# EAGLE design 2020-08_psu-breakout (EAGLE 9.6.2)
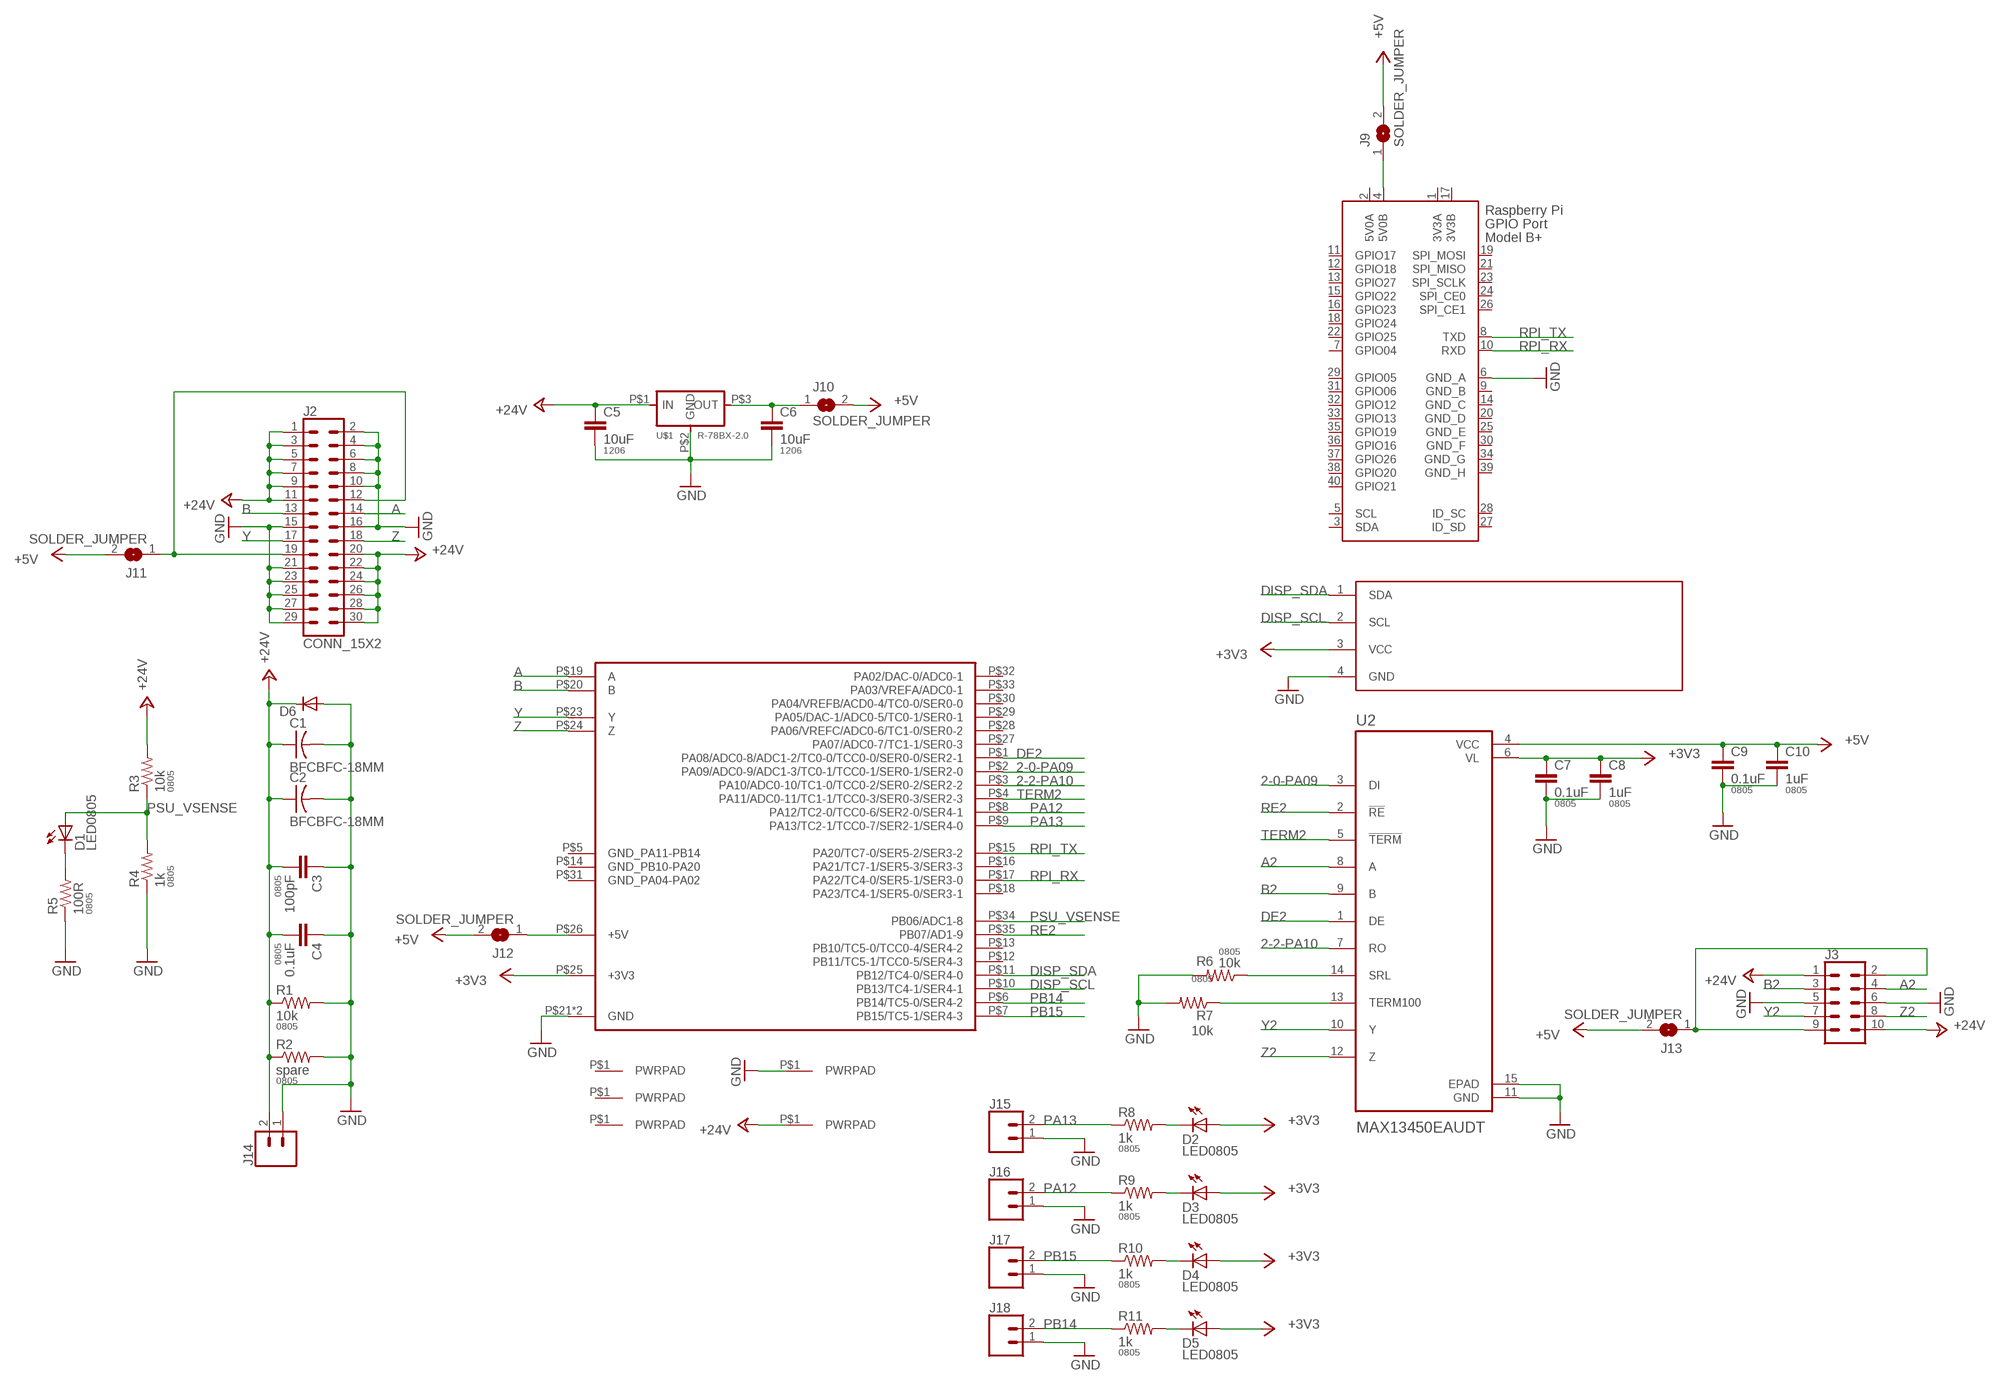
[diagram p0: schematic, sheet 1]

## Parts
C1  BFCBFC-18MM  [BFC-18MM-7-5MM]
C2  BFCBFC-18MM  [BFC-18MM-7-5MM]
C3  100pF  CAP0805  [0805]
C4  0.1uF  CAP0805  [0805]
C5  10uF  CAP1206  [1206]
C6  10uF  CAP1206  [1206]
C7  0.1uF  CAP0805  [0805]
C8  1uF  CAP0805  [0805]
C9  0.1uF  CAP0805  [0805]
C10  1uF  CAP0805  [0805]
D1  LED0805  [LED0805]
D2  LED0805  [LED0805]
D3  LED0805  [LED0805]
D4  LED0805  [LED0805]
D5  LED0805  [LED0805]
D6  DIODESMA403D  [SMA-403D]
J1  I2C_OLED_MODULE  [I2C_MODULE_0.91INCH_PLANAR]
J2  CONN_15X2  [2X15-SHROUDED]
J3  CONN_05X2SHD_LOCK  [2X5-SHROUDED_LOCK]
J4  PWRPADM3-SKINNY  [PWRPAD_3-25MM-SKINNY]
J5  PWRPADM3-SKINNY  [PWRPAD_3-25MM-SKINNY]
J6  PWRPADM3-SKINNY  [PWRPAD_3-25MM-SKINNY]
J7  PWRPADSOLDER  [SOLDER_ON]
J8  PWRPADSOLDER  [SOLDER_ON]
J9  SOLDER_JUMPER  [SOLDER_JUMPER]
J10  SOLDER_JUMPER  [SOLDER_JUMPER]
J11  SOLDER_JUMPER  [SOLDER_JUMPER]
J12  SOLDER_JUMPER  [SOLDER_JUMPER]
J13  SOLDER_JUMPER  [SOLDER_JUMPER]
J14  CONN_02LOCK  [1X02_LOCK]
J15  CONN_02LOCK  [1X02_LOCK]
J16  CONN_02LOCK  [1X02_LOCK]
J17  CONN_02LOCK  [1X02_LOCK]
J18  CONN_02LOCK  [1X02_LOCK]
R1  10k  RESISTOR0805-RES  [0805]
R2  spare  RESISTOR0805-RES  [0805]
R3  10k  RESISTOR0805-RES  [0805]
R4  1k  RESISTOR0805-RES  [0805]
R5  100R  RESISTOR0805-RES  [0805]
R6  10k  RESISTOR0805-RES  [0805]
R7  10k  RESISTOR0805-RES  [0805]
R8  1k  RESISTOR0805-RES  [0805]
R9  1k  RESISTOR0805-RES  [0805]
R10  1k  RESISTOR0805-RES  [0805]
R11  1k  RESISTOR0805-RES  [0805]
U1  UCBUS_MODULE  [UCBUS_MODULE]
U2  MAX13450EAUDT  [SOP65P637X110-14N]
U$1  R-78BX-2.0  [R-78BX-2.0]
X1  RASPI_BOARD_B+#_F  [RASPI_BOARD_B+_FULL]

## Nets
2-0-PA09: U1.P$2(PA09/ADC0-9/ADC1-3/TC0-1/TCC0-1/SER0-1/SER2-0) U2.3(DI)
2-2-PA10: U1.P$3(PA10/ADC0-10/TC1-0/TCC0-2/SER0-2/SER2-2) U2.7(RO)
+3V3: C7.1 C8.1 D2.1(A) D3.1(A) D4.1(A) D5.1(A) J1.3(VCC) U1.P$25(+3V3) U2.6(VL)
+5V: C9.1 C10.1 J9.2 J10.2 J11.2 J12.2 J13.2 U2.4(VCC)
+24V: C1.P$2 C2.P$2 C3.2 C4.2 C5.1 D6.P$1(C) J2.1 J2.3 J2.5 J2.7 J2.9 J2.11 J2.20 J2.22 J2.24 J2.26 J2.28 J2.30 J3.1 J3.10 J8.P$1(PWRPAD) J14.2 R1.1 R2.1 R3.2 U$1.P$1(IN)
A: J2.14 U1.P$19(A)
A2: J3.4 U2.8(A)
B: J2.13 U1.P$20(B)
B2: J3.3 U2.9(B)
DE2: U1.P$1(PA08/ADC0-8/ADC1-2/TC0-0/TCC0-0/SER0-0/SER2-1) U2.1(DE)
DISP_SCL: J1.2(SCL) U1.P$10(PB13/TC4-1/SER4-1)
DISP_SDA: J1.1(SDA) U1.P$11(PB12/TC4-0/SER4-0)
GND: C1.P$1 C2.P$1 C3.1 C4.1 C5.2 C6.2 C7.2 C8.2 C9.2 C10.2 D6.P$2(A) J1.4(GND) J2.2 J2.4 J2.6 J2.8 J2.10 J2.15 J2.16 J2.21 J2.23 J2.25 J2.27 J2.29 J3.5 J3.6 J7.P$1(PWRPAD) J14.1 J15.1 J16.1 J17.1 J18.1 R1.2 R2.2 R4.1 R5.1 R6.2 R7.2 U1.P$21(GND) U1.P$22(GND) U2.11(GND) U2.15(EPAD) U$1.P$2(GND) X1.6(GND_A)
N$1: D3.2(C) R9.2
N$2: D1.2(C) R5.2
N$3: D2.2(C) R8.2
N$4: D4.2(C) R10.2
N$5: C6.1 J10.1 U$1.P$3(OUT)
N$6: J9.1 X1.4(5V0B)
N$7: R7.1 U2.13(TERM100)
N$8: R6.1 U2.14(SRL)
N$9: D5.2(C) R11.2
N$10: J3.2 J3.9 J13.1
N$11: J2.12 J2.19 J11.1
N$12: J12.1 U1.P$26(+5V)
PA12: J16.2 R9.1 U1.P$8(PA12/TC2-0/TCC0-6/SER2-0/SER4-1)
PA13: J15.2 R8.1 U1.P$9(PA13/TC2-1/TCC0-7/SER2-1/SER4-0)
PB14: J18.2 R11.1 U1.P$6(PB14/TC5-0/SER4-2)
PB15: J17.2 R10.1 U1.P$7(PB15/TC5-1/SER4-3)
PSU_VSENSE: D1.1(A) R3.1 R4.2 U1.P$34(PB06/ADC1-8)
RE2: U1.P$35(PB07/AD1-9) U2.2(!RE)
RPI_RX: U1.P$17(PA22/TC4-0/SER5-1/SER3-0) X1.10(RXD)
RPI_TX: U1.P$15(PA20/TC7-0/SER5-2/SER3-2) X1.8(TXD)
TERM2: U1.P$4(PA11/ADC0-11/TC1-1/TCC0-3/SER0-3/SER2-3) U2.5(!TERM)
Y: J2.17 U1.P$23(Y)
Y2: J3.7 U2.10(Y)
Z: J2.18 U1.P$24(Z)
Z2: J3.8 U2.12(Z)
Unconnected: J4.P$1(PWRPAD) J5.P$1(PWRPAD) J6.P$1(PWRPAD) U1.P$5(GND_PA11-PB14) U1.P$12(PB11/TC5-1/TCC0-5/SER4-3) U1.P$13(PB10/TC5-0/TCC0-4/SER4-2) U1.P$14(GND_PB10-PA20) U1.P$16(PA21/TC7-1/SER5-3/SER3-3) U1.P$18(PA23/TC4-1/SER5-0/SER3-1) U1.P$27(PA07/ADC0-7/TC1-1/SER0-3) U1.P$28(PA06/VREFC/ADC0-6/TC1-0/SER0-2) U1.P$29(PA05/DAC-1/ADC0-5/TC0-1/SER0-1) U1.P$30(PA04/VREFB/ACD0-4/TC0-0/SER0-0) U1.P$31(GND_PA04-PA02) U1.P$32(PA02/DAC-0/ADC0-1) U1.P$33(PA03/VREFA/ADC0-1) X1.3(SDA) X1.5(SCL) X1.7(GPIO04) X1.11(GPIO17) X1.12(GPIO18) X1.13(GPIO27) X1.15(GPIO22) X1.16(GPIO23) X1.18(GPIO24) X1.19(SPI_MOSI) X1.21(SPI_MISO) X1.22(GPIO25) X1.23(SPI_SCLK) X1.24(SPI_CE0) X1.26(SPI_CE1) X1.27(ID_SD) X1.28(ID_SC) X1.29(GPIO05) X1.31(GPIO06) X1.32(GPIO12) X1.33(GPIO13) X1.35(GPIO19) X1.36(GPIO16) X1.37(GPIO26) X1.38(GPIO20) X1.40(GPIO21)

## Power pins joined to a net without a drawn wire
3V3A: X1.1(3V3A)
3V3B: X1.17(3V3B)
5V0A: X1.2(5V0A)
GND_B: X1.9(GND_B)
GND_C: X1.14(GND_C)
GND_D: X1.20(GND_D)
GND_E: X1.25(GND_E)
GND_F: X1.30(GND_F)
GND_G: X1.34(GND_G)
GND_H: X1.39(GND_H)

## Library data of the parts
C1 C2 = power:BFC
C3 C4 C7-C10 = passives:CAP: Capacitor; PACKAGE: 0805
C5 C6 = passives:CAP: Capacitor; PACKAGE: 1206
D1-D5 = lights:LED: LED
D6 = passives:DIODE: DIODE
J1 = lights:I2C_OLED_MODULE
J2 = SparkFun-Connectors:CONN_15X2
J3 = SparkFun-Connectors:CONN_05X2: Multi connection point. Often used as Generic Header-pin footprint for 0.1 inch spaced/style header connections For AVR SPI programming port, see special device with nice symbol: "AVR_SPI_PROG_5x2.dev" You can populate with any combo of single row headers, but if you'd like an exact match, check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; PROD_ID: CONN-08671; SF_ID: PRT-08506
J4-J8 = connector:PWRPAD
J9-J13 = connector:SOLDER_JUMPER
J14-J18 = SparkFun-Connectors:CONN_02: Multi connection point. Often used as Generic Header-pin footprint for 0.1 inch spaced/style header connections
R1-R11 = passives:RESISTOR: Resistor; PACKAGE: 0805
U1 = connector:UCBUS_MODULE
U2 = comm:MAX13450EAUDT; DESCRIPTION: 1/1 Transceiver Full RS422, RS485 14-TSSOP-EP; DIGI-KEY_PART_NUMBER: MAX13450EAUD+T-ND; DIGIKEY-PURCHASE-URL: https://snapeda.com/shop?store=DigiKey&id=694117; MF: Maxim Integrated; MP: MAX13450EAUD+; PACKAGE: TSSOP-14 Maxim
U$1 = power:R-78BX-2.0
X1 = raspberrypi_bastelstube_v13:RASPI_BOARD_B+#: Raspberry Pi GPIO connector with markings for the outer dimensions of the Raspberry Pi board model B+ with different sets of drill holes or mounting pads All pins connected

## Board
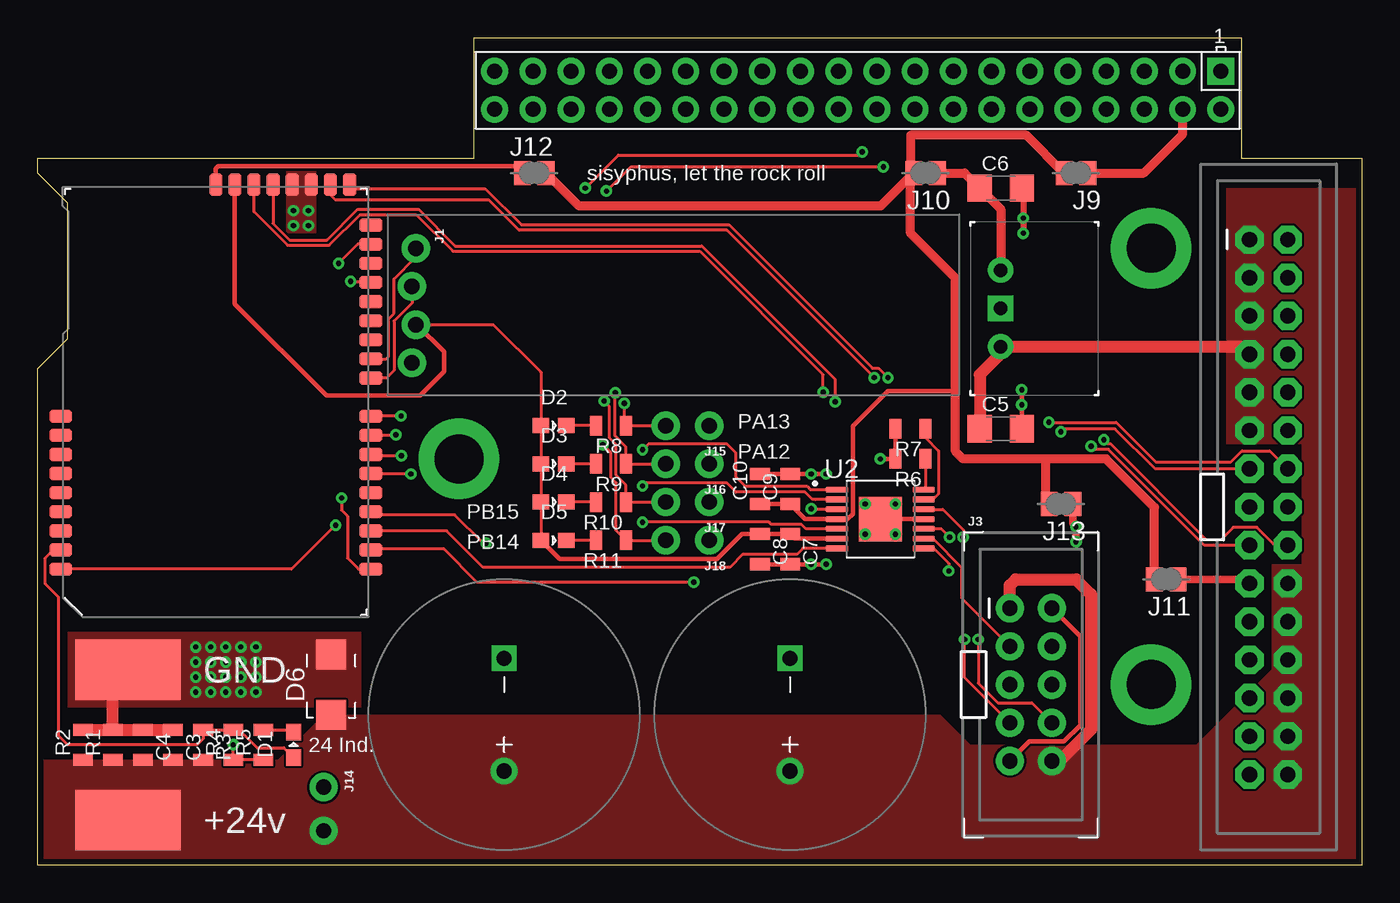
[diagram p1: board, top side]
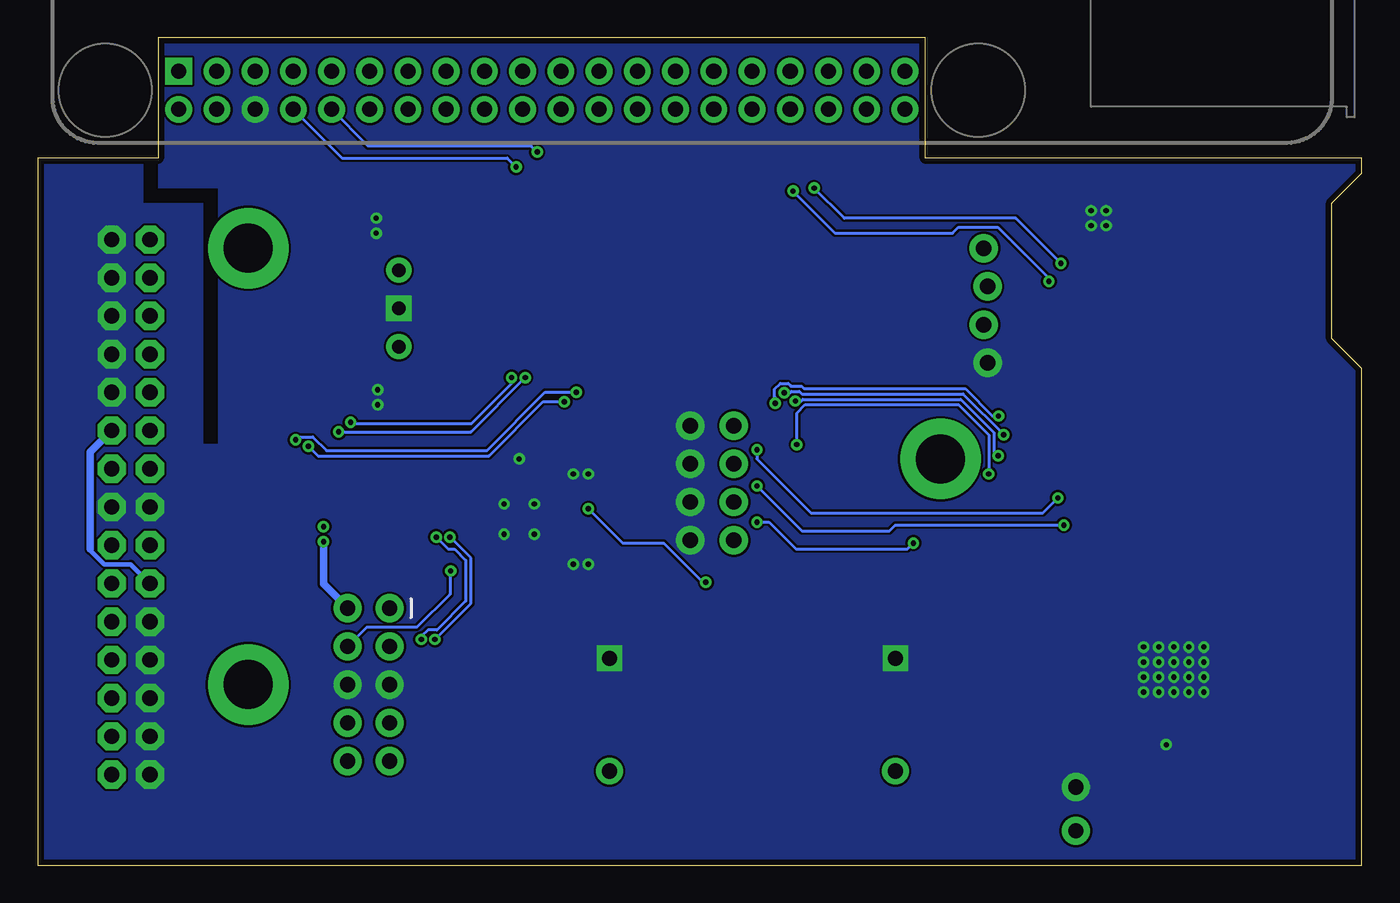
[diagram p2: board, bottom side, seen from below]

Size 88 x 55 mm. Coordinates in mm from the lower left corner, seen from the top.
Outline: 0,0 0,33 2,35 2,44 0,46 0,47 29,47 29,55 80,55 80,47 88,47 88,0 0,0
Copper layers (1*16): Top 0.035mm / dielectric 1.5mm / Bottom 0.035mm
Design rules "default *": minimum track width 6mil, minimum drill 0.35mm, track to track 6mil, track to pad 6mil, pad to pad 6mil, via to via 6mil, smd to smd 0mil, copper to edge 16mil, drill to drill 6mil, minimum pad ring 10mil, minimum via ring 8mil, stop-mask expansion 4mil, vias tented up to drill 35mil, thermal gap 10mil

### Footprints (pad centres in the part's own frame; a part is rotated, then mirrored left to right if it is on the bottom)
BFC-18MM-7-5MM = drill 1 pad 1.676 square: P$1 -3.75,0 | drill 1 pad 1.778: P$2 3.75,0
0805 = smd 0.8 x 1.3: 1 -1,0; 2 1,0
1206 = smd 1.6 x 1.8: 1 -1.4,0; 2 1.4,0
LED0805 = smd 1.1 x 1: 1 -0.85,0; 2 0.85,0
SMA-403D = smd 2 x 2: P$1 -2,0; P$2 2,0
I2C_MODULE_0.91INCH_PLANAR = drill 1.016 pad 1.88: 1 0,0.127; 2 2.54,-0.127; 3 5.08,0.127; 4 7.62,-0.127
2X15-SHROUDED = drill 1.016 pad 1.88 octagon: 1 -1.27,17.78; 2 1.27,17.78; 3 -1.27,15.24; 4 1.27,15.24; 5 -1.27,12.7; 6 1.27,12.7; 7 -1.27,10.16; 8 1.27,10.16; 9 -1.27,7.62; 10 1.27,7.62; 11 -1.27,5.08; 12 1.27,5.08; 13 -1.27,2.54; 14 1.27,2.54; 15 -1.27,0; 16 1.27,0; 17 -1.27,-2.54; 18 1.27,-2.54; 19 -1.27,-5.08; 20 1.27,-5.08; 21 -1.27,-7.62; 22 1.27,-7.62; 23 -1.27,-10.16; 24 1.27,-10.16; 25 -1.27,-12.7; 26 1.27,-12.7; 27 -1.27,-15.24; 28 1.27,-15.24; 29 -1.27,-17.78; 30 1.27,-17.78
2X5-SHROUDED_LOCK = drill 1.016 pad 1.88: 1 -1.397,5.08; 2 1.397,5.08; 3 -1.397,2.54; 4 1.397,2.54; 5 -1.397,0; 6 1.397,0; 7 -1.397,-2.54; 8 1.397,-2.54; 9 -1.397,-5.08; 10 1.397,-5.08
PWRPAD_3-25MM-SKINNY = drill 3.25 pad 5.35: P$1 0,0
SOLDER_ON = smd 4 x 7: P$1 0,0
SOLDER_JUMPER = smd 1.118 x 1.6: 1 -0.787,0; 2 0.787,0
1X02_LOCK = drill 1.016 pad 1.88: 1 -0.178,0; 2 2.718,0
UCBUS_MODULE = smd 0.889 x 1.524: P$1 3.175,-0.152; P$2 4.445,-0.152; P$3 5.715,-0.152; P$4 6.985,-0.152; P$5 8.255,-0.152; P$6 9.525,-0.152; P$7 10.795,-0.152; P$8 12.065,-0.152; P$9 13.335,-0.152; P$10 15.875,-0.152; P$11 17.145,-0.152; P$12 18.415,-0.152; P$13 19.685,-0.152; P$14 20.955,-0.152; P$15 22.225,-0.152; P$16 23.495,-0.152; P$17 24.765,-0.152; P$18 26.035,-0.152; P$27 13.335,20.472; P$28 12.065,20.472; P$29 10.795,20.472; P$30 9.525,20.472; P$31 8.255,20.472; P$32 6.985,20.472; P$33 5.715,20.472; P$34 4.445,20.472; P$35 3.175,20.472 | smd 1.524 x 0.889: P$19 28.727,1.27; P$20 28.727,2.54; P$21 28.727,3.81; P$22 28.727,5.08; P$23 28.727,6.35; P$24 28.727,7.62; P$25 28.727,8.89; P$26 28.727,10.16
SOP65P637X110-14N = smd 1.48 x 0.41: 1 -2.875,1.95; 2 -2.875,1.3; 3 -2.875,0.65; 4 -2.875,0; 5 -2.875,-0.65; 6 -2.875,-1.3; 7 -2.875,-1.95; 8 2.875,-1.95; 9 2.875,-1.3; 10 2.875,-0.65; 11 2.875,0; 12 2.875,0.65; 13 2.875,1.3; 14 2.875,1.95 | smd 2.85 x 2.95: 15 0,0
R-78BX-2.0 = drill 0.9 pad 1.676: P$1 -2.54,0; P$3 2.54,0 | drill 0.9 pad 1.676 square: P$2 0,0
RASPI_BOARD_B+_FULL = drill 1 pad 1.778 square: 1 8.37,51.23 | drill 1 pad 1.778: 2 8.37,53.77; 3 10.91,51.23; 4 10.91,53.77; 5 13.45,51.23; 6 13.45,53.77; 7 15.99,51.23; 8 15.99,53.77; 9 18.53,51.23; 10 18.53,53.77; 11 21.07,51.23; 12 21.07,53.77; 13 23.61,51.23; 14 23.61,53.77; 15 26.15,51.23; 16 26.15,53.77; 17 28.69,51.23; 18 28.69,53.77; 19 31.23,51.23; 20 31.23,53.77; 21 33.77,51.23; 22 33.77,53.77; 23 36.31,51.23; 24 36.31,53.77; 25 38.85,51.23; 26 38.85,53.77; 27 41.39,51.23; 28 41.39,53.77; 29 43.93,51.23; 30 43.93,53.77; 31 46.47,51.23; 32 46.47,53.77; 33 49.01,51.23; 34 49.01,53.77; 35 51.55,51.23; 36 51.55,53.77; 37 54.09,51.23; 38 54.09,53.77; 39 56.63,51.23; 40 56.63,53.77

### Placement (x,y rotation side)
C1  31,10 270 top
C2  50,10 270 top
C3  9,8 270 top
C4  7,8 270 top
C5  64,29 0 top
C6  64,45 0 top
C7  50,21 270 top
C8  48,21 270 top
C9  50,25 90 top
C10  48,25 90 top
D1  17,8 90 top
D2  34.29,29.21 0 top
D3  34.29,26.67 0 top
D4  34.29,24.13 0 top
D5  34.29,21.59 0 top
D6  19.5,12 90 top
J1  25,41 270 top
J2  81.8,23.8 0 top
J3  66,12 0 top
J4  28,27 0 top
J5  74,41 0 top
J6  74,12 0 top
J7  6,13 270 top
J8  6,3 270 top
J9  69,46 180 top
J10  59,46 180 top
J11  75,19 180 top
J12  33,46 0 top
J13  68,24 180 top
J14  19,5 270 top
J15  44.45,29.21 180 top
J16  44.45,26.67 180 top
J17  44.45,24.13 180 top
J18  44.45,21.59 180 top
R1  5,8 90 top
R2  3,8 90 top
R3  11,8 270 top
R4  13,8 90 top
R5  15,8 90 top
R6  58,27 180 top
R7  58,29 180 top
R8  38.1,29.21 180 top
R9  38.1,26.67 180 top
R10  38.1,24.13 180 top
R11  38.1,21.59 180 top
U1  22,16.5 90 top
U2  56,23 0 top
U$1  64,37 90 top
X1  87,104 180 top

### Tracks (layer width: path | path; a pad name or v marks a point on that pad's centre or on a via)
2-0-PA09  (via drill 0.35)
  Top 0.203: U2.3 51.43,23.65 v51.4,23.68 | v43.6,18.8 29.2,18.8 27,21 22.21,21 U1.P$2
  Bottom 0.203: v51.4,23.68 49.12,21.4 46.4,21.4 43.8,18.8 v43.6,18.8
2-2-PA10
  Top 0.203: U2.7 50.85,21.05 50.45,20.65 46.85,20.65 46,19.8 29.6,19.8 27.18,22.21 U1.P$3
+3V3
  Top 0.203: D5.1 D4.1 D3.1 D2.1 33.44,32.76 30.28,35.92 25.2,35.92 J1.3
  Top 0.305: U2.6 50.3,21.7 C7.1 C8.1 46.8,22 45.14,20.34 34.69,20.34 D5.1 | U1.P$25 13.11,37.29 19.2,31.2 25.4,31.2 27,32.8 27,34.12 25.2,35.92
+5V
  Top 0.305: C10.1 C9.1 51,23 U2.4 53.82,23 54.17,23.35 54.17,29.17 56.5,31.5 61,31.5
  Top 0.61: J9.2 65.71,48.5 58,48.5 58,46.21 J10.2 | J10.2 56.01,43.8 35.99,43.8 J12.2 | J11.2 74.21,23.79 71,27 67,27 | 67,27 67,24.21 J13.2 | 67,27 61.5,27 61,27.5 61,31.5 61,39 58,42 58,45.79 J10.2
+24V
  Top 0.813: J3.1 64.6,18.6 65,19 69,19 70,18 70,9 67.92,6.92 J3.10 | C5.1 62.6,32.6 64,34 U$1.P$1 80.03,34.46 J2.7
  pour Top (rank 2, no thermals): -2,7 16,7 19,10 60,10 62,8 77,8 82,13 82,20 84,20 84,28 79,28 79,45 90,45 90,-2 -2,-2
A  (via drill 0.35)
  Top 0.203: U1.P$19 20.77,45.23 21.04,44.96 29.75,44.96 32.15,42.56 45.95,42.56 55.47,33.03 55.86,33.03 56.49,32.4 v56.51,32.4 | J2.14 81.88,27.53 80.04,27.53 79.3,26.8 74.3,26.8 71.67,29.43 v67.2,29.43
  Bottom 0.203: v56.51,32.4 56.51,31.99 59.15,29.36 67.12,29.36 v67.2,29.43
A2  (via drill 0.35)
  Top 0.203: U2.8 59.55,21.05 60.55,20.05 v60.55,19.55
  Bottom 0.203: v60.55,19.55 60.6,19.5 60.6,18 62.8,15.8 66.14,15.8 J3.4
B  (via drill 0.35)
  Top 0.203: J2.13 74.26,26.34 71.6,29 68.2,29 v68,28.8 | v55.6,32.4 45.8,42.2 32,42.2 30,44.2 19.8,44.2 19.4,44.6 19.4,45.17 U1.P$20
  Bottom 0.203: v68,28.8 59.2,28.8 v55.6,32.4
B2
  Top 0.203: U2.9 59.49,21.71 61.4,19.8 61.4,17.74 J3.3
DE2  (via drill 0.35)
  Top 0.203: U2.1 51.35,24.95 51.15,25.16 47.04,25.16 46.4,25.8 46.4,27.4 45.8,28 40.6,28 v40.2,27.6 | v20.2,24.4 20.2,23.6 20.6,23.2 20.6,20.4 21.32,19.68 U1.P$1
  Bottom 0.203: v40.2,27.6 40.2,27 36.6,23.4 21.2,23.4 v20.2,24.4
DISP_SCL
  Top 0.203: J1.2 24.87,37.35 23.68,36.16 23.68,32.88 23.18,32.38 U1.P$10
DISP_SDA
  Top 0.203: U1.P$11 23.17,33.65 23.32,33.8 23.32,36.31 23.68,36.66 23.68,38.95 25.13,40.4 J1.1
GND  (via drill 0.35)
  Top 0.152: U2.15 v55,22
  Top 0.203: R5.1 R4.1 v13,8
  Top 0.305: C8.2 C7.2 v51.4,20 v52.4,20 | C10.2 C9.2 v51.4,26 v52.4,26 | R7.2 R6.2 v56,27 | U2.11 57.2,23 57,22.8 v57,22 | C5.2 v65.4,30.6 v65.4,31.6
  Top 0.406: C6.2 65.5,44.9 v65.5,43 v65.5,42
  Top 0.813: R2.2 R1.2 | R1.2 C4.1 C3.1 | J7.P$1 5,12 R1.2
  other vias: 10.5,11.5 10.5,12.5 10.5,13.5 10.5,14.5 11.5,14.5 11.5,13.5 11.5,12.5 11.5,11.5 12.5,14.5 12.5,13.5 12.5,12.5 12.5,11.5 13.5,11.5 13.5,12.5 13.5,13.5 13.5,14.5 14.5,14.5 14.5,13.5 14.5,12.5 14.5,11.5 17,43.5 18,43.5 18,42.5 17,42.5 55,24 57,24
  pour Bottom (rank 2, no thermals): -1,-1 89,-1 89,56 81,56 81,44 77,44 77,28 76,28 76,45 80,45 80,56 -1,56
  pour Top (rank 2, no thermals): 2,10.5 21.5,10.5 21.5,15.5 2,15.5
  pour Top (rank 2, no thermals): 16.5,47.5 16.5,42 18.5,42 18.5,47.5
N$1
  Top 0.203: R9.2 D3.2
N$2
  Top 0.203: R5.2 16.85,9 D1.2
N$3
  Top 0.203: R8.2 D2.2
N$4
  Top 0.203: R10.2 D4.2
N$5
  Top 0.61: J10.1 61.6,46 C6.1 64,43.6 U$1.P$3
N$6
  Top 0.61: J9.1 73.5,46 76.09,48.59 X1.4
N$7
  Top 0.203: R7.1 59,28.41 59.87,27.54 59.87,24.67 59.5,24.3 U2.13
N$8
  Top 0.203: R6.1 59,25.07 U2.14
N$9
  Top 0.203: R11.2 D5.2
N$10  (via drill 0.35)
  Top 0.305: J3.9 65.9,8.21 68.21,8.21 69.29,9.29 69.29,15.19 J3.2
  Top 0.508: J13.1 68.79,22.71 v69,22.5 v69,21.5
  Bottom 0.508: J3.2 69,18.68 v69,21.5
N$11
  Top 0.508: J11.1 80.25,19 J2.19
  Bottom 0.305: 84.5,21 84.5,20.93 83.57,20 81.81,20 J2.19
  Bottom 0.508: J2.12 84.5,27.45 84.5,21
N$12
  Top 0.305: U1.P$26 11.84,46.28 12,46.44 31.77,46.44 J12.1
PA12  (via drill 0.35)
  Top 0.203: J16.2 R9.1 39.1,27.8 38.36,28.55 38.36,31.36 v38.39,31.39 | v23.8,28.6 23.77,28.57 U1.P$8
  Bottom 0.203: v38.39,31.39 38,31.39 37.91,31.48 37.38,31.48 37.22,31.31 26.5,31.31 v23.8,28.61 v23.8,28.6
PA13  (via drill 0.35)
  Top 0.203: J15.2 R8.1 38.99,29.32 v38.99,30.7 | v24.15,29.85 24.14,29.84 U1.P$9
  Bottom 0.203: v38.99,30.7 38.99,31.09 39.02,31.13 39.02,31.65 38.65,32.02 38.13,32.02 37.94,31.84 37.23,31.84 37.07,31.67 26.36,31.67 24.54,29.85 v24.15,29.85
PB14  (via drill 0.35)
  Top 0.203: J18.2 R11.1 38.45,22.24 38.45,25.41 38.09,25.77 38.09,27.41 v37.55,27.95 | v24.79,26 22.18,26 U1.P$6
  Bottom 0.203: v37.55,27.95 37.55,30.05 37,30.6 26.8,30.6 24.79,28.59 v24.79,26
PB15  (via drill 0.35)
  Top 0.203: J17.2 R10.1 39.1,25.26 38.45,25.91 38.45,27.95 38,28.4 38,30.49 v37.65,30.85 | v24.16,27.2 22.25,27.2 U1.P$7
  Bottom 0.203: v37.65,30.85 37.26,30.85 37.15,30.96 26.65,30.96 24.44,28.74 24.44,27.48 v24.16,27.2
PSU_VSENSE
  Top 0.203: D1.1 16.35,7.8 14.6,7.8 13.4,9 R4.2 R3.1 11,8.4 10.6,8 2,8 1.4,8.6 1.4,17.8 0.51,18.69 0.51,20.4 1.05,20.95 U1.P$34
RE2  (via drill 0.35)
  Top 0.203: U2.2 51.68,24.3 51.66,24.32 51.48,24.32 51,24.8 46.4,24.8 45.8,25.4 40.4,25.4 v40.2,25.2 | v19.8,22.6 16.88,19.68 U1.P$35
  Bottom 0.203: v40.2,25.2 37.2,22.2 31.4,22.2 31,22.6 v19.8,22.6
RPI_RX  (via drill 0.35)
  Top 0.203: U1.P$17 21.27,41.27 v20,40 | v36.4,45 38.6,47.2 54.6,47.2 v54.8,47.4
  Bottom 0.203: v20,40 23,43 34.4,43 v36.4,45 | v54.8,47.4 55.2,47.8 66.04,47.8 X1.10
RPI_TX  (via drill 0.35)
  Top 0.203: v56.2,46.4 39.4,46.4 v37.8,44.8 | v20.8,38.8 22.08,38.8 U1.P$15
  Bottom 0.203: X1.8 67.78,47 56.8,47 v56.2,46.4 | v37.8,44.8 35,42 27.2,42 26.8,42.4 24.2,42.4 20.8,39 v20.8,38.8
TERM2  (via drill 0.35)
  Top 0.203: U2.5 51.06,22.35 50.76,22.65 48.75,22.65 48.6,22.8 v40.2,22.8 | v29.8,21.4 29.6,21.4 27.71,23.29 22.35,23.29 U1.P$4
  Bottom 0.203: v29.8,21.4 30.2,21 37.6,21 39.4,22.8 v40.2,22.8
Y  (via drill 0.35)
  Top 0.203: J2.17 77.53,21.26 71.16,27.64 70.2,27.64 v70,27.84 | U1.P$23 15.65,42.65 16.75,41.56 19.23,41.56 21.27,43.59 25.31,43.59 27.75,41.16 44.15,41.16 53,32.3 v53,30.8
  Bottom 0.203: v70,27.84 69.36,27.2 58,27.2 54.4,30.8 v53,30.8
Y2  (via drill 0.35)
  Top 0.203: J3.7 61.6,12.46 v61.6,15 | v60.6,21.8 60.05,22.35 U2.10
  Bottom 0.203: v61.6,15 59.2,17.4 59.2,20.4 v60.6,21.8
Z  (via drill 0.35)
  Top 0.203: J2.18 82.22,21.26 81.02,22.45 79.45,22.45 78.62,21.62 77.68,21.62 71.3,27.99 71.13,27.99 v70.85,28.27 | v52.2,31.43 52.2,32.6 44,40.8 27.6,40.8 25.17,43.23 21.41,43.23 19.38,41.2 16.6,41.2 14.38,43.42 U1.P$24
  Bottom 0.203: v70.85,28.27 70.65,28.47 69.71,28.47 68.8,27.56 58.15,27.56 54.27,31.43 v52.2,31.43
Z2  (via drill 0.35)
  Top 0.203: U2.12 60.15,23.65 61.51,22.29 v61.51,21.8 | v62.51,15 62.51,12.09 63.8,10.8 66.06,10.8 J3.8
  Bottom 0.203: v61.51,21.8 60.71,21 60.3,21 59.56,20.25 59.56,17.55 61.47,15.63 62.06,15.63 62.51,15.19 v62.51,15

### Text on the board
tPlace: sisyphus, let the rock roll | PA13 | PA12 | PB15 | PB14 | GND | 24 Ind. | +24v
